FUNCTION_BLOCK Absolute_Move_DUT

VAR_IN_OUT
    SD_SMD_IO: DUT_AMCI_Stepper;
END_VAR	

VAR_INPUT
	
FB_Target_Position: DINT;
    FB_Programmed_Speed: UDINT;
	FB_Acceleration: UINT;
	FB_Deceleration: UINT;
	FB_Jerk: UINT;
	
	
END_VAR

VAR_OUTPUT
	Enable: BOOL :=FALSE;
	Error: BOOL :=TRUE;
		
END_VAR

VAR	
	I_Command_Word_1: UINT;
	
END_VAR
VAR // added by the converter: edge detectors and wires of the graphical bodies
    _w1, _w2 : BOOL;
END_VAR

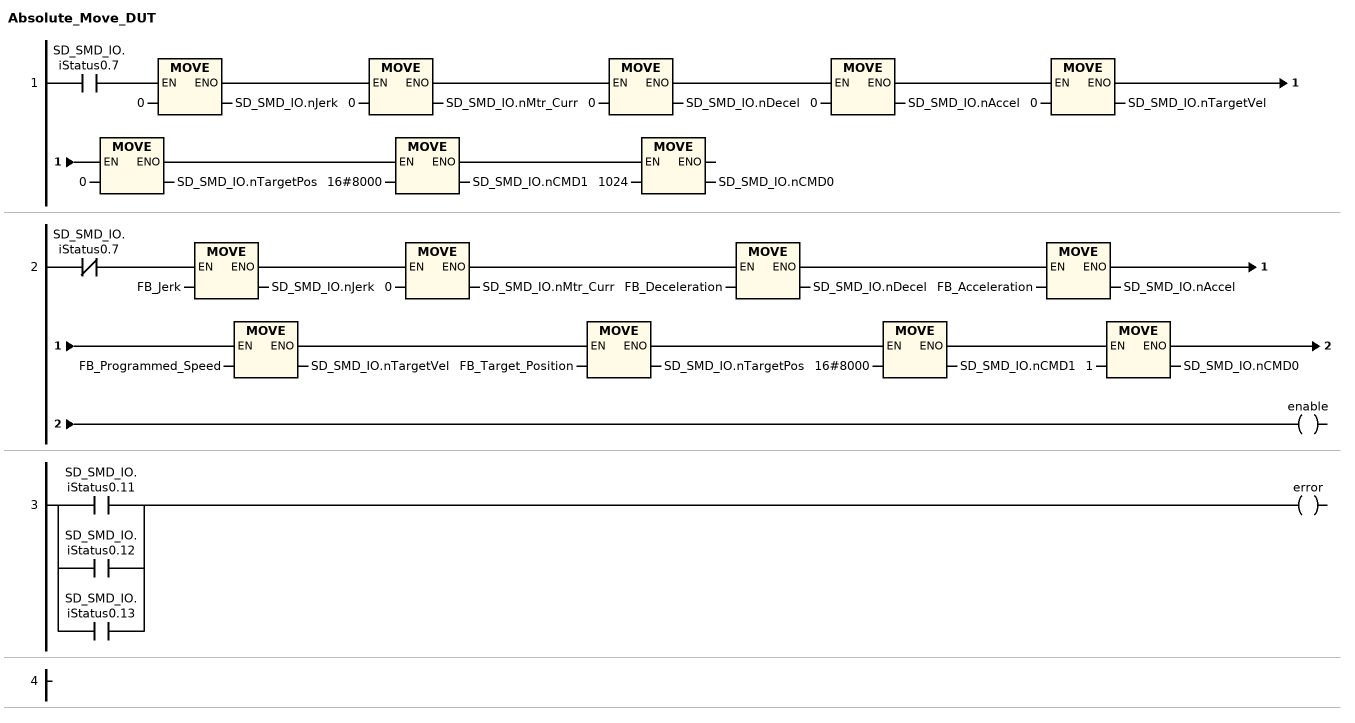
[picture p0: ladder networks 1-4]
// NETWORK 1
_w1 := SD_SMD_IO.iStatus0.7;
IF _w1 THEN SD_SMD_IO.nJerk := 0; END_IF
IF _w1 THEN SD_SMD_IO.nMtr_Curr := 0; END_IF
IF _w1 THEN SD_SMD_IO.nDecel := 0; END_IF
IF _w1 THEN SD_SMD_IO.nAccel := 0; END_IF
IF _w1 THEN SD_SMD_IO.nTargetVel := 0; END_IF
IF _w1 THEN SD_SMD_IO.nTargetPos := 0; END_IF
IF _w1 THEN SD_SMD_IO.nCMD1 := 16#8000; END_IF
IF _w1 THEN SD_SMD_IO.nCMD0 := 1024; END_IF

// NETWORK 2
_w2 := NOT SD_SMD_IO.iStatus0.7;
IF _w2 THEN SD_SMD_IO.nJerk := FB_Jerk; END_IF
IF _w2 THEN SD_SMD_IO.nMtr_Curr := 0; END_IF
IF _w2 THEN SD_SMD_IO.nDecel := FB_Deceleration; END_IF
IF _w2 THEN SD_SMD_IO.nAccel := FB_Acceleration; END_IF
IF _w2 THEN SD_SMD_IO.nTargetVel := FB_Programmed_Speed; END_IF
IF _w2 THEN SD_SMD_IO.nTargetPos := FB_Target_Position; END_IF
IF _w2 THEN SD_SMD_IO.nCMD1 := 16#8000; END_IF
IF _w2 THEN SD_SMD_IO.nCMD0 := 1; END_IF
enable := _w2;

// NETWORK 3
error := SD_SMD_IO.iStatus0.11 OR SD_SMD_IO.iStatus0.12 OR SD_SMD_IO.iStatus0.13;

// NETWORK 4

END_FUNCTION_BLOCK
